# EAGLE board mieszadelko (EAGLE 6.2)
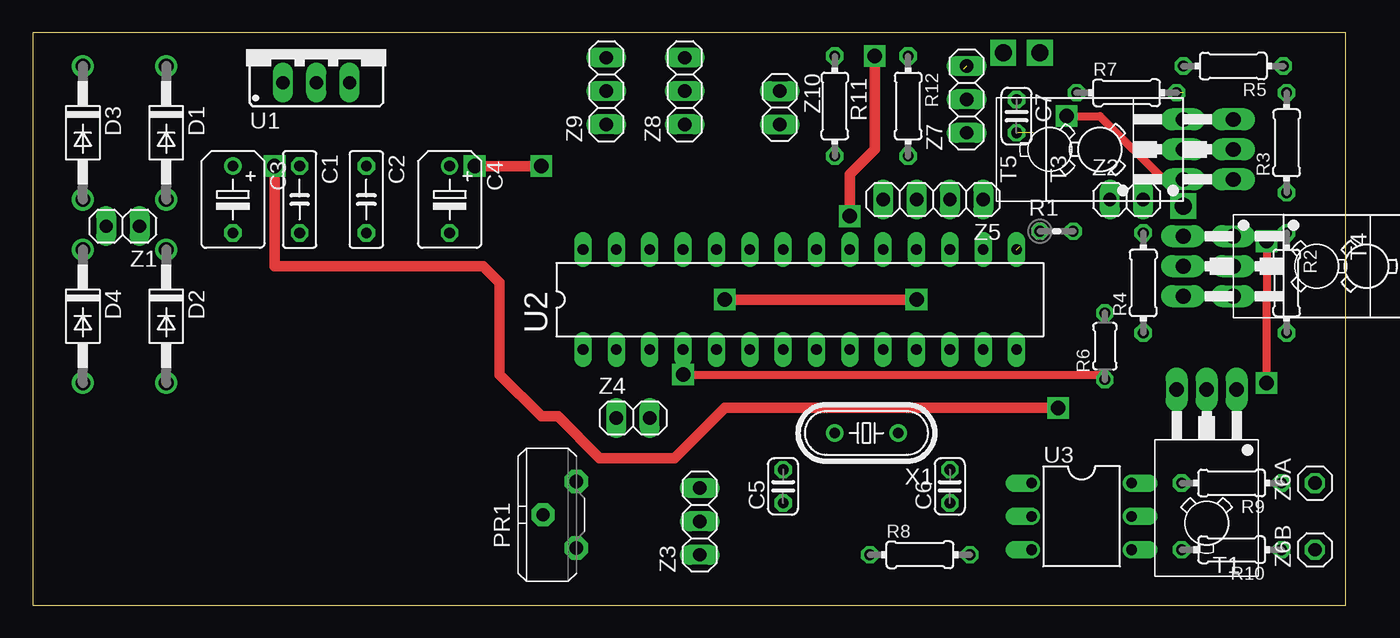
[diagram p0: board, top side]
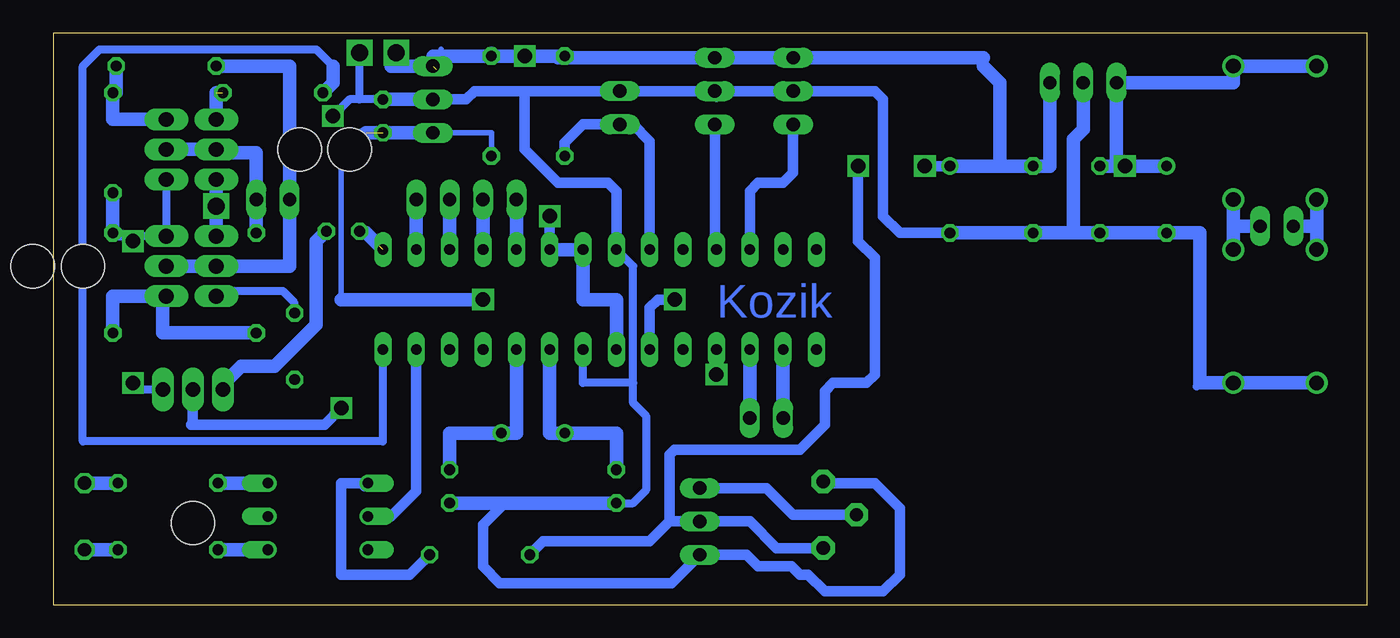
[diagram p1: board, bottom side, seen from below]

Size 100 x 43.57 mm. Coordinates in mm from the lower left corner, seen from the top.
Outline: 0,0 100,0 100,43.57 0,43.57 0,0
Copper layers (1*16): Top 0.035mm / dielectric 1.5mm / Bottom 0.035mm
Design rules: minimum track width 10mil, minimum drill 24mil, track to track 8mil, track to pad 8mil, pad to pad 8mil, via to via 8mil, smd to smd 8mil, copper to edge 40mil, drill to drill 8mil, minimum pad ring 10mil, minimum via ring 8mil, stop-mask expansion 4mil, vias tented up to drill 0mil, thermal gap 10mil

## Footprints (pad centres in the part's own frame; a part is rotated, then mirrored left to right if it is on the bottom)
C050-025X075 = drill 0.813 octagon: 1 -2.54,0; 2 2.54,0
B45181B = drill 0.813: + -2.54,0 | drill 0.813 octagon: - 2.54,0
C025-024X044 = drill 0.813 octagon: 1 -1.27,0; 2 1.27,0
DO41-10 = drill 1.118: A 5.08,0; C -5.08,0
PT-10S = drill 1.016 pad 1.778 octagon: 1 -2.54,-1.27; 2 2.54,-1.27; 3 0,1.27
0204V = drill 0.813 octagon: 1 -1.27,0; 2 1.27,0
0204/7 = drill 0.813 octagon: 1 -3.81,0; 2 3.81,0
0204/5 = drill 0.813 octagon: 1 -2.54,0; 2 2.54,0
TO126 = drill 1.118 long: 1 -2.286,-5.08; 2 0,-5.08; 3 2.286,-5.08 | hole 3.302: 0,5.08
78XXS = drill 1.016 long: GND 0,-2.54; IN -2.54,-2.54; OUT 2.54,-2.54
DIL28-3 = drill 0.813 long: 1 -16.51,-3.81; 2 -13.97,-3.81; 3 -11.43,-3.81; 4 -8.89,-3.81; 5 -6.35,-3.81; 6 -3.81,-3.81; 7 -1.27,-3.81; 8 1.27,-3.81; 9 3.81,-3.81; 10 6.35,-3.81; 11 8.89,-3.81; 12 11.43,-3.81; 13 13.97,-3.81; 14 16.51,-3.81; 15 16.51,3.81; 16 13.97,3.81; 17 11.43,3.81; 18 8.89,3.81; 19 6.35,3.81; 20 3.81,3.81; 21 1.27,3.81; 22 -1.27,3.81; 23 -3.81,3.81; 24 -6.35,3.81; 25 -8.89,3.81; 26 -11.43,3.81; 27 -13.97,3.81; 28 -16.51,3.81
DIL06 = drill 0.813 offset: 1 -2.54,-3.81; 2 0,-3.81; 3 2.54,-3.81; 4 2.54,3.81; 5 0,3.81; 6 -2.54,3.81
HC49/S = drill 0.813: 1 -2.413,0; 2 2.413,0
1X02 = drill 1.016 long: 1 -1.27,0; 2 1.27,0
1X03 = drill 1.016 long: 1 -2.54,0; 2 0,0; 3 2.54,0
1X04 = drill 1.016 long: 1 -3.81,0; 2 -1.27,0; 3 1.27,0; 4 3.81,0
1X01 = drill 1.016 octagon: 1 0,0

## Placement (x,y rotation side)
C1  [C050-025X075]  20.32,30.88 270 top
C2  [C050-025X075]  25.4,30.88 270 top
C3  [B45181B]  15.24,30.88 270 top
C4  [B45181B]  31.75,30.88 270 top
C5  [C025-024X044]  57.15,9.04 90 top
C6  [C025-024X044]  69.85,9.04 90 top
C7  [C025-024X044]  74.93,37.23 270 top
D1  1N4004  [DO41-10]  10.16,35.96 270 top
D2  1N4004  [DO41-10]  10.16,21.99 270 top
D3  1N4004  [DO41-10]  3.81,35.96 270 top
D4  1N4004  [DO41-10]  3.81,21.99 270 top
PR1  [PT-10S]  40.13,6.88 90 top
R1  [0204V]  77.98,28.47 0 top
R2  [0204/7]  95.5,24.53 270 top
R3  [0204/7]  95.5,35.2 90 top
R4  [0204/7]  84.58,24.53 90 top
R5  [0204/7]  91.44,41.04 180 top
R6  [0204/5]  81.66,19.7 90 top
R7  [0204/7]  83.31,39.01 0 top
R8  [0204/7]  67.56,3.83 0 top
R9  [0204/7]  91.31,9.29 180 top
R10  [0204/7]  91.31,4.21 180 top
R11  [0204/7]  61.09,37.99 270 top
R12  [0204/7]  66.67,37.99 270 top
T1  BD139  [TO126]  89.41,11.32 180 top
T2  BD140  [TO126]  96.52,25.8 270 top
T3  BD140  [TO126]  86.36,34.69 90 top
T4  BD139  [TO126]  92.71,25.8 270 top
T5  BD139  [TO126]  82.55,34.69 90 top
U1  [78XXS]  21.59,42.31 0 top
U2  MEGA8-P  [DIL28-3]  58.42,23.26 0 top
U3  MOC3031M  [DIL06]  79.88,6.75 270 top
X1  [HC49/S]  63.5,13.1 180 top
Z1  [1X02]  6.86,28.85 180 top
Z2  [1X02]  83.31,30.88 0 top
Z3  [1X03]  50.8,6.37 90 top
Z4  [1X02]  45.72,14.24 0 top
Z5  [1X04]  68.58,30.88 180 top
Z6A  [1X01]  97.66,9.29 90 top
Z6B  [1X01]  97.66,4.21 90 top
Z7  [1X03]  71.12,38.5 90 top
Z8  [1X03]  49.66,39.13 90 top
Z9  [1X03]  43.69,39.13 90 top
Z10  [1X02]  56.9,37.87 270 top

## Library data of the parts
C1-C7 PR1 R1-R12 = rcl
D1-D4 = diode
T1 T4 T5 = transistor-npn
T2 T3 = transistor-pnp
U1 = v-reg-2
U2 = atmel
U3 = optocoupler
X1 = crystal
Z1 Z2 Z10 = pinhead1
Z3-Z5 Z6A Z6B Z7-Z9 = pinhead

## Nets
+5V: C2.1 C4.+ PR1.1 R8.1 R11.1 R12.1 U1.OUT U2.7 U2.20 U2.21 Z3.2 Z7.3 Z8.3 Z9.3
GND: C1.2 C2.2 C3.- C4.- C5.1 C6.1 C7.1 D2.A D4.A PR1.2 T4.1 T5.1 U1.GND U2.8 U2.22 Z3.1 Z7.2 Z8.2 Z9.2 Z10.1
GRZALKA: U2.13 U3.2
M1: R6.1 U2.4
M2: R7.1 U2.14
N$3: U2.19 Z5.4
N$4: R2.1 R3.1 T1.1 T2.1 T3.1
N$5: R10.2 U3.4
N$6: R9.2 U3.6
N$7: C5.2 U2.9 X1.2
N$8: C6.2 U2.10 X1.1
N$9: U2.18 Z5.3
N$10: U2.17 Z5.2
N$11: U2.16 Z5.1
N$12: R5.2 T2.2 T4.2 Z2.1
N$13: R8.2 U3.1
N$14: R7.2 T5.3
N$17: R6.2 T4.3
N$18: R9.1 Z6A.1
N$19: D1.A D2.C Z1.1
N$20: R2.2 R4.1 T2.3
N$21: R3.2 R5.1 T3.3
N$22: R4.2 T3.2 T5.2 Z2.2
N$23: D3.A D4.C Z1.2
N$24: R10.1 Z6B.1
N$25: U2.2 Z4.1
N$26: U2.3 Z4.2
N$27: PR1.3 Z3.3
N$34: R1.2 T1.3
NASTAWA_PREDKOSC: U2.26 Z9.1
NASTAWA_TEMPERATURY: U2.25 Z8.1
OBROTY: C7.2 R12.2 U2.6 Z7.1
ODLICZANIE: U2.5
PWM: R1.1 U2.15
TEMPERATURA: R11.2 U2.23 Z10.2
VCC: C1.1 C3.+ D1.C D3.C T1.2 U1.IN

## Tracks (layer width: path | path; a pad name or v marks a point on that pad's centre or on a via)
+5V  (via drill 1.1)  (1 unrouted)
  Top 0.813: v62.23,29.61 62.23,32.79 64.14,34.69 v64.14,41.8 | v38.73,33.42 35.56,33.42 34.92,33.42 v33.66,33.42
  Bottom 0.406: 70.87,40.79 70.48,40.79 70.48,42.31 | 66.67,42.31 R12.1 66.67,41.68 | Z8.3 50.16,41.68 | 29.21,41.68 29.21,41.04 | 61.09,41.68 R11.1 60.96,41.8 60.96,41.68 61.09,41.68
  Bottom 0.813: PR1.1 44.96,4.34 46.99,6.37 Z3.2 53.09,6.37 | 53.09,6.37 54.61,4.84 62.74,4.84 R8.1 | U2.20 v62.23,29.61 | 53.09,6.37 53.09,11.45 52.7,11.83 43.18,11.83 41.27,13.73 41.27,16.27 40.64,16.91 38.1,16.91 37.47,17.55 37.47,26.44 38.73,27.71 v38.73,33.42 | C4.+ v33.66,33.42
  Bottom 1.016: U2.20 U2.21 59.69,23.26 57.15,23.26 U2.7 | 27.94,33.42 C2.1 24.13,33.42 U1.OUT | 27.94,33.42 C4.+ | 29.21,41.04 27.94,39.77 27.94,33.42 | 29.21,41.68 Z9.3 50.16,41.68 61.59,41.68 61.59,41.8 | R11.1 61.59,41.8 | 61.59,41.8 v64.14,41.8 R12.1 71.12,41.8 Z7.3 74.3,41.04 74.3,41.68
GND  (via drill 1.1, 1.3)
  Top 0.61: v78.74,37.23 81.28,37.23 86.36,32.15 87.38,32.15 T5.1
  Bottom 0.406: 50.8,39.13 50.16,39.13 Z8.2 49.53,39.13 49.53,38.5 | 64.14,39.13 64.77,39.13
  Bottom 0.61: U2.22 55.88,25.8 55.88,16.91 | 55.88,16.91 59.69,16.91 U2.8 | C7.1 76.71,38.5 | 76.71,38.5 76.71,41.29 | C5.1 55.88,7.77 54.86,8.78 54.86,14.37 55.88,15.39 55.88,16.91 | 12.95,16.66 12.7,16.91 | 76.71,38.5 77.47,38.5 v78.74,37.23
  Bottom 0.813: PR1.2 41.27,9.29 37.47,9.29 35.56,7.38 35.56,2.3 36.83,1.04 41.27,1.04 42.55,2.3 43.18,2.3 43.81,2.94 46.35,2.94 47.24,3.83 Z3.1 52.96,1.67 66.04,1.67 67.31,2.94 67.31,6.12 65.66,7.77 C5.1 | C4.- 35.56,28.34 36.83,29.61 36.83,38.5 37.47,39.13 Z9.2 50.16,39.13 | 50.8,39.13 Z10.1 64.77,39.13 67.94,39.13 68.58,38.5 71.75,38.5 | U2.22 57.15,31.51 57.78,32.15 61.59,32.15 64.14,34.69 64.14,39.13
  Bottom 1.016: C5.1 C6.1 | D4.A D2.A 12.7,16.91 12.7,28.34 C3.- C1.2 22.61,28.34 | 22.61,28.34 C2.2 C4.- | U1.GND 21.59,36.21 22.35,35.45 22.35,28.59 22.61,28.34 | T4.1 v87.63,30.37 T5.1 | Z7.2 71.75,38.5 C7.1
GRZALKA
  Bottom 0.813: U2.13 72.39,8.66 74.3,6.75 U3.2
M1  (via drill 1.1)
  Top 0.61: v49.53,17.55 81.28,17.55 R6.1
  Bottom 0.61: U2.4 v49.53,17.55
M2
  Bottom 0.61: 78.74,41.04 80.01,42.31 96.52,42.31 97.79,41.04 97.79,12.47 74.93,12.47 U2.14
  Bottom 1.016: R7.1 78.74,39.77 78.74,41.04
N$3
  Bottom 1.016: U2.19 Z5.4
N$4  (via drill 1.1)
  Top 0.61: v93.98,16.91 93.98,20.72 93.98,23.26 v93.98,27.71
  Bottom 0.61: T1.1 93.47,16.4 v93.98,16.91 | T3.1 T2.1 94.36,28.09 | R2.1 95.25,28.09 94.36,28.09 | 94.36,28.09 v93.98,27.71
  Bottom 1.016: R3.1 R2.1 95.25,28.34
N$5
  Bottom 1.016: U3.4 R10.2
N$6
  Bottom 1.016: U3.6 R9.2
N$7
  Bottom 1.016: U2.9 62.23,13.1 X1.2 57.15,13.1 C5.2
N$8
  Bottom 1.016: U2.10 64.77,13.1 X1.1 69.85,13.1 C6.2
N$9
  Bottom 1.016: U2.18 Z5.3
N$10
  Bottom 1.016: U2.17 Z5.2
N$11
  Bottom 1.016: U2.16 Z5.1
N$12
  Bottom 1.016: T2.2 T4.2 82.04,25.8 Z2.1 82.04,41.04 R5.2
N$13
  Bottom 0.813: 76.33,9.04 75.82,9.04 75.56,9.29 U3.1 | U3.1 76.2,9.29 | U3.1 78.11,9.29 78.11,2.3 72.9,2.3 R8.2
N$14  (1 unrouted)
  Bottom 1.016: 87.63,39.01 T5.3
N$17
  Bottom 0.61: R6.2 81.66,23.01 82.55,23.9 87.25,23.9 T4.3
  Bottom 1.016: T4.3 87.38,23.26
N$18
  Bottom 1.016: R9.1 Z6A.1
N$19
  Bottom 1.016: Z1.1 10.16,28.85 | 10.16,28.85 D1.A | D2.C 10.16,28.85
N$20
  Bottom 1.016: R2.2 95.5,23.51 T2.3 91.69,23.51 91.69,20.72 R4.1
N$21
  Bottom 1.016: R5.1 95.25,39.01 R3.2 95.5,36.98 T3.3
N$22
  Bottom 1.016: T3.2 T5.2 87.63,34.44 84.58,34.44 Z2.2 R4.2
N$23
  Bottom 1.016: D4.C 3.81,28.85 | 3.81,28.85 D3.A | 3.81,28.85 Z1.2
N$24
  Bottom 1.016: R10.1 Z6B.1
N$25
  Bottom 1.016: Z4.1 U2.2
N$26
  Bottom 1.016: Z4.2 U2.3
N$27
  Bottom 0.813: Z3.3 45.72,8.91 43.69,6.88 PR1.3
N$28  (via drill 1.3)
  other vias: 73.91,42.06
N$29  (via drill 1.3)
  other vias: 76.71,42.06
N$34
  Bottom 1.016: R1.2 80.01,27.71 80.01,21.35 83.19,18.18 85.72,18.18 87.12,16.78 T1.3
NASTAWA_PREDKOSC
  Bottom 0.813: Z9.1 43.69,32.91 44.45,32.15 46.35,32.15 46.99,31.51 U2.26
NASTAWA_TEMPERATURY
  Bottom 0.406: U2.25 49.66,27.07
  Bottom 0.813: 49.66,27.07 Z8.1
OBROTY  (via drill 1.1)  (1 unrouted)
  Top 0.813: v52.7,23.26 v67.31,23.26
  Bottom 0.406: R12.2 66.67,35.96 Z7.1 | 78.11,34.69 78.11,23.26
  Bottom 0.813: U2.6 54.61,22.62 53.98,23.26 v52.7,23.26
  Bottom 1.016: 78.11,23.26 v67.31,23.26 | 78.11,34.69 76.2,35.96 Z7.1
PWM  (1 unrouted)
  Bottom 1.016: U2.15 76.2,28.34 76.58,28.34 R1.1
TEMPERATURA
  Bottom 0.813: U2.23 54.61,35.32 55.88,36.6 Z10.2 59.69,36.6 61.09,35.2 R11.2
VCC  (via drill 1.1)
  Top 0.813: v78.11,15.01 52.7,15.01 48.9,11.2 43.18,11.2 40.01,14.37 38.73,14.37 35.56,17.55 35.56,24.53 34.29,25.8 18.41,25.8 v18.41,33.42
  Bottom 0.813: T1.2 89.41,13.86 89.53,13.73 79.38,13.73 v78.11,15.01
  Bottom 1.016: D3.C D1.C 10.16,39.77 U1.IN 19.05,33.42 | C3.+ v18.41,33.42 19.05,33.42 | 19.05,33.42 C1.1

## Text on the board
Bottom: Kozik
